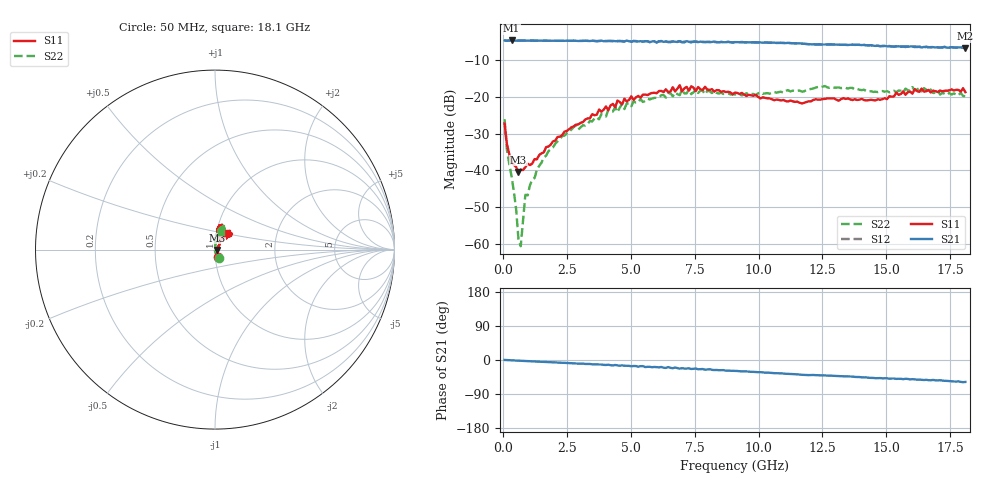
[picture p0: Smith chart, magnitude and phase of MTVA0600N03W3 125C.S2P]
! Network Analyzer HP8720D.06.14 Serial No. US36140669
!  8 Jul 2005  10:17:47
! Frequency  S11  S21  S12  S22
# HZ  S  DB R 50
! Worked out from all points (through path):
!   201 points, 50 MHz to 18.1 GHz, reference 50 ohm
!   highest |S21| = -4.59 dB at 320.8 MHz (marker M1); lowest = -6.7 dB at 18.1 GHz (marker M2)
!   group delay of S21, straight-line fit = 8.96 ps
!   lowest |S11| = -40.4 dB at 591.5 MHz (marker M3), VSWR 1.02, Z = 50.9 - j0.194 ohm
!   |S11| at or under -10 dB: start of sweep to end of sweep
!   |S22| runs from -60.6 to -17.0 dB; largest |S21 - S12| = 0.023
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5e7  -27.21 -68.9  -4.60 0.1  -4.62 0.3  -26.03 -66.0
1.4025e8  -32.85 -56.8  -4.67 -0.2  -4.66 -0.3  -34.33 -81.5
3.2075e8  -37.79 -38.2  -4.59 -0.8  -4.62 -0.8  -41.55 -85.5
5.0125e8  -39.04 -17.9  -4.65 -1.7  -4.63 -1.7  -50.51 -95.4
5.915e8  -40.43 -11.5  -4.62 -1.6  -4.65 -1.7  -58.65 -127.4
6.8175e8  -39.75 -4.0  -4.65 -2.1  -4.65 -2.2  -60.62 146.9
8.6225e8  -39.10 10.8  -4.64 -2.6  -4.66 -2.7  -46.63 134.7
9.525e8  -38.13 16.0  -4.66 -2.9  -4.64 -3.0  -46.78 104.2
1.3135e9  -36.98 32.4  -4.65 -4.2  -4.65 -4.1  -39.80 87.8
2.30625e9  -30.38 44.8  -4.69 -7.3  -4.68 -7.3  -30.64 84.6
3.1185e9  -26.82 57.1  -4.69 -9.5  -4.72 -9.9  -27.68 89.2
4.11125e9  -23.64 62.3  -4.71 -12.4  -4.76 -13.4  -23.41 83.3
4.47225e9  -20.94 60.1  -4.82 -14.2  -4.71 -13.6  -24.12 87.6
4.65275e9  -21.99 61.1  -4.87 -14.2  -4.74 -15.1  -21.89 87.2
6.09675e9  -18.37 68.8  -4.87 -19.4  -4.78 -19.4  -20.09 78.2
6.909e9  -16.79 74.6  -4.76 -22.7  -4.87 -21.5  -19.48 73.3
7.54075e9  -18.36 73.5  -4.97 -22.7  -4.84 -24.8  -17.77 78.2
9.075e9  -18.80 81.9  -5.06 -28.7  -5.03 -28.8  -19.26 70.1
1.21435e10  -20.80 68.1  -5.64 -39.5  -5.59 -39.7  -17.70 71.2
1.512175e10  -19.79 46.2  -6.20 -49.2  -6.07 -48.9  -18.71 75.7
1.602425e10  -19.08 43.4  -6.24 -50.6  -6.37 -52.4  -17.30 70.2
1.81e10  -18.66 54.0  -6.70 -57.9  -6.81 -58.8  -19.78 72.2
